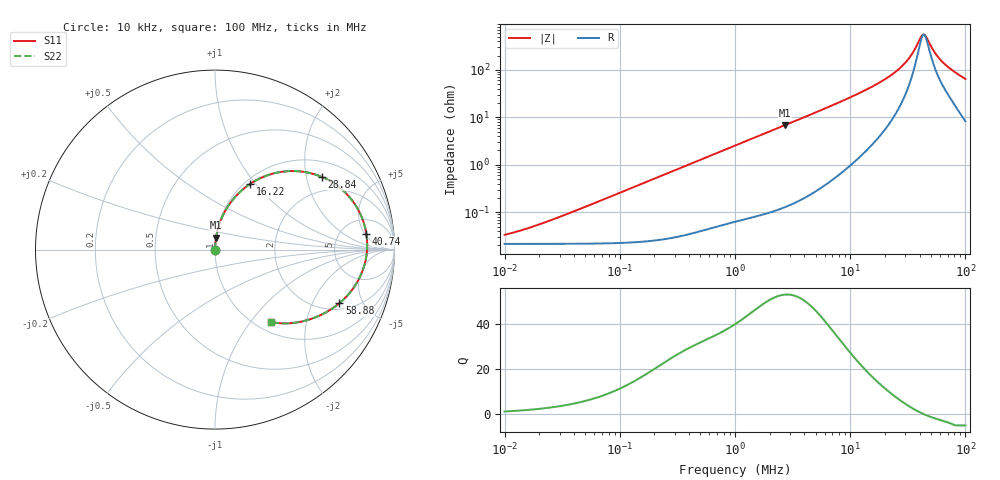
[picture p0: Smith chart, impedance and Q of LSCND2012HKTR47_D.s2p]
! LSCND2012HKTR47_D  S-PARAMETER MODEL  ( Standard Model )
! Model Generated by TAIYO YUDEN Corporation (http://www.ty-top.com)
! Version 1.0
! TAIYO YUDEN Control No. 210402
! Copyright(c) 2021 TAIYO YUDEN CO.,LTD. All Rights Reserved.
! Product Description (link to TY-COMPAS)
! https://ds.yuden.co.jp/TYCOMPAS/or/detail?pn=LSCND2012HKTR47MD&u=M
! Products Name : Inductors
! Characteristics :
!  Inductance : 0.47 [uH] , SRF(min) : - [Hz] , DC Resistance(max) : 26 [mOhm]
!  Rated Current : Saturation  4.8 [A] (dL = 30 [%]), Temp Rise  4.0 [A] (dT = 40 [degC])
!  Case Size : 2.0 x 1.2 / 0.079 x 0.047 [mm/inch] , Thickness : 0.8 / 0.031 [mm/inch]
!  (Conditions: Temperature = 25 [degC] , DC Bias Current = 0 [A])
! External Node Assignments :
!  1  o---GGG---o  2
! GND o---------o GND
! Frequency Range : 10kHz  -  100MHz  [ 402 STEP ]
# MHz S RI R 50
! Freq[MHz].  S11 Real  S11 Imag  S21 Real  S21 Imag  S12 Real  S12 Imag  S22 Real  S22 Imag
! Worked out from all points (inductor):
!   401 points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, 10 kHz to 100 MHz, reference 50 ohm
!   read as one part in series: L = 407 nH near 25.7 kHz
!   highest Q = 53.1 at 2.692 MHz (marker M1), where L = 398 nH
!   self-resonance near 43.64 MHz
!   S11 on the Smith chart (normalised r, x): 10 kHz: 1.00, +0.00; 16.22 MHz: 1.06, +0.93; 28.84 MHz: 1.47, +2.48; 40.74 MHz: 9, +5; 58.88 MHz: 2.35, -3.26; 100 MHz: 1.16, -1.27
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0.01  0.000215 0.000256  0.9998 -0.000256  0.9998 -0.000256  0.000215 0.000256
0.018621  0.000216 0.000476  0.9998 -0.000476  0.9998 -0.000476  0.000216 0.000476
0.046774  0.000219 0.0012  0.9998 -0.0012  0.9998 -0.0012  0.000219 0.0012
0.218776  0.000292 0.00558  0.9997 -0.00558  0.9997 -0.00558  0.000292 0.00558
1  0.00126 0.0251  0.9987 -0.0251  0.9987 -0.0251  0.00126 0.0251
2.691535  0.00576 0.0668  0.9942 -0.0668  0.9942 -0.0668  0.00576 0.0668
4.677351  0.016 0.1155  0.984 -0.1155  0.984 -0.1155  0.016 0.1155
10  0.0722 0.2411  0.9278 -0.2411  0.9278 -0.2411  0.0722 0.2411
16.2181  0.1948 0.3654  0.8052 -0.3654  0.8052 -0.3654  0.1948 0.3654
21.87762  0.3593 0.4314  0.6407 -0.4314  0.6407 -0.4314  0.3593 0.4314
25.11886  0.4693 0.4361  0.5307 -0.4361  0.5307 -0.4361  0.4693 0.4361
28.84032  0.5972 0.4041  0.4028 -0.4041  0.4028 -0.4041  0.5972 0.4041
31.62278  0.6843 0.3536  0.3157 -0.3536  0.3157 -0.3536  0.6843 0.3536
34.67368  0.7623 0.2765  0.2377 -0.2765  0.2377 -0.2765  0.7623 0.2765
40.73803  0.8432 0.089  0.1568 -0.089  0.1568 -0.089  0.8432 0.089
42.65795  0.8481 0.0295  0.1519 -0.0295  0.1519 -0.0295  0.8481 0.0295
44.66836  0.8444 -0.0295  0.1556 0.0295  0.1556 0.0295  0.8444 -0.0295
52.48075  0.7749 -0.2089  0.2251 0.2089  0.2251 0.2089  0.7749 -0.2089
58.88437  0.6935 -0.2982  0.3065 0.2982  0.3065 0.2982  0.6935 -0.2982
66.06934  0.6052 -0.3566  0.3948 0.3566  0.3948 0.3566  0.6052 -0.3566
75.85776  0.5013 -0.3965  0.4987 0.3965  0.4987 0.3965  0.5013 -0.3965
100  0.3136 -0.4038  0.6864 0.4038  0.6864 0.4038  0.3136 -0.4038
